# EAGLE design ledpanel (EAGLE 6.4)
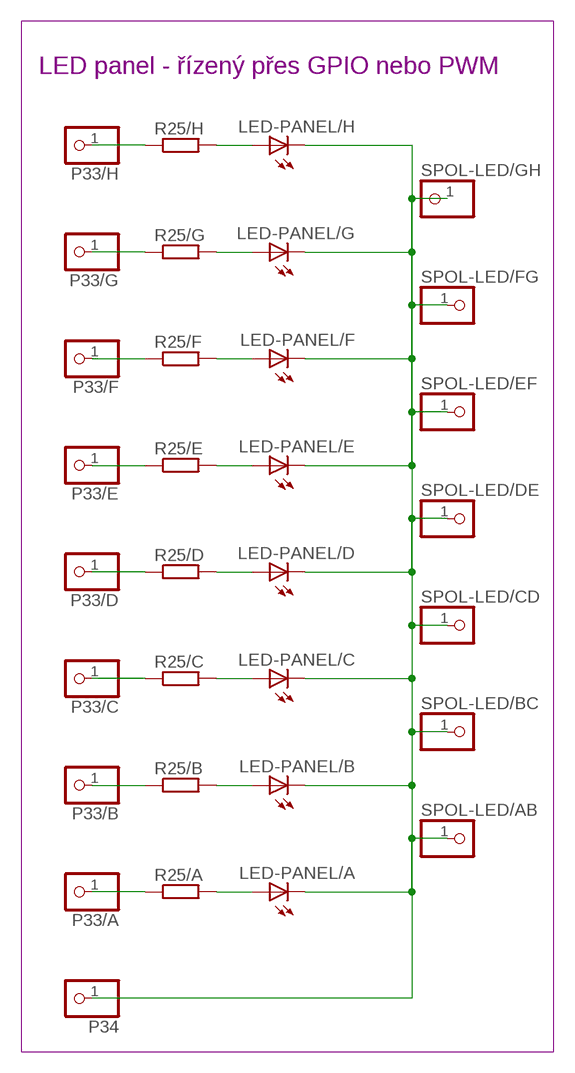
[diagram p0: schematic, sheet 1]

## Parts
LED-PANEL/A  TLLG4400  [LED3MM]
LED-PANEL/B  TLLG4400  [LED3MM]
LED-PANEL/C  TLLG4400  [LED3MM]
LED-PANEL/D  TLLG4400  [LED3MM]
LED-PANEL/E  TLLG4400  [LED3MM]
LED-PANEL/F  TLLG4400  [LED3MM]
LED-PANEL/G  TLLG4400  [LED3MM]
LED-PANEL/H  TLLG4400  [LED3MM]
P33/A  HEADER-1X1  [1X01_OVAL]
P33/B  HEADER-1X1  [1X01_OVAL]
P33/C  HEADER-1X1  [1X01_OVAL]
P33/D  HEADER-1X1  [1X01_OVAL]
P33/E  HEADER-1X1  [1X01_OVAL]
P33/F  HEADER-1X1  [1X01_OVAL]
P33/G  HEADER-1X1  [1X01_OVAL]
P33/H  HEADER-1X1  [1X01_OVAL]
P34  HEADER-1X1  [1X01_OVAL]
R25/A  1k  R-EU_M0805  [M0805]
R25/B  1k  R-EU_M0805  [M0805]
R25/C  1k  R-EU_M0805  [M0805]
R25/D  1k  R-EU_M0805  [M0805]
R25/E  1k  R-EU_M0805  [M0805]
R25/F  1k  R-EU_M0805  [M0805]
R25/G  1k  R-EU_M0805  [M0805]
R25/H  1k  R-EU_M0805  [M0805]
SPOL-LED/AB  PINHD-1X1  [1X01]
SPOL-LED/BC  PINHD-1X1  [1X01]
SPOL-LED/CD  PINHD-1X1  [1X01]
SPOL-LED/DE  PINHD-1X1  [1X01]
SPOL-LED/EF  PINHD-1X1  [1X01]
SPOL-LED/FG  PINHD-1X1  [1X01]
SPOL-LED/GH  PINHD-1X1  [1X01]

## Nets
LED-SPOL: LED-PANEL/A.K(C) LED-PANEL/B.K(C) LED-PANEL/C.K(C) LED-PANEL/D.K(C) LED-PANEL/E.K(C) LED-PANEL/F.K(C) LED-PANEL/G.K(C) LED-PANEL/H.K(C) P34.1 SPOL-LED/AB.1 SPOL-LED/BC.1 SPOL-LED/CD.1 SPOL-LED/DE.1 SPOL-LED/EF.1 SPOL-LED/FG.1 SPOL-LED/GH.1
PRA: P33/A.1 R25/A.1
PRB: P33/B.1 R25/B.1
PRC: P33/C.1 R25/C.1
PRD: P33/D.1 R25/D.1
PRE: P33/E.1 R25/E.1
PRF: P33/F.1 R25/F.1
PRG: P33/G.1 R25/G.1
PRH: P33/H.1 R25/H.1
RLA: LED-PANEL/A.A R25/A.2
RLB: LED-PANEL/B.A R25/B.2
RLC: LED-PANEL/C.A R25/C.2
RLD: LED-PANEL/D.A R25/D.2
RLE: LED-PANEL/E.A R25/E.2
RLF: LED-PANEL/F.A R25/F.2
RLG: LED-PANEL/G.A R25/G.2
RLH: LED-PANEL/H.A R25/H.2

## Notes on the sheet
- LED panel - řízený přes GPIO nebo PWM

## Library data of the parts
LED-PANEL/A LED-PANEL/B LED-PANEL/C LED-PANEL/D LED-PANEL/E LED-PANEL/F LED-PANEL/G LED-PANEL/H = led:TLLG4400: Low Current (2mA) LED 3 mm Tinted Diffused Package color GREEN; MF: VISHAY SEMICONDUCTOR; OC_FARNELL: 1612435
P33/A P33/B P33/C P33/D P33/E P33/F P33/G P33/H P34 = nonolith:HEADER-1X1: PIN HEADER
R25/A R25/B R25/C R25/D R25/E R25/F R25/G R25/H = resistor:R-EU_: RESISTOR, European symbol
SPOL-LED/AB SPOL-LED/BC SPOL-LED/CD SPOL-LED/DE SPOL-LED/EF SPOL-LED/FG SPOL-LED/GH = pinhead:PINHD-1X1: PIN HEADER

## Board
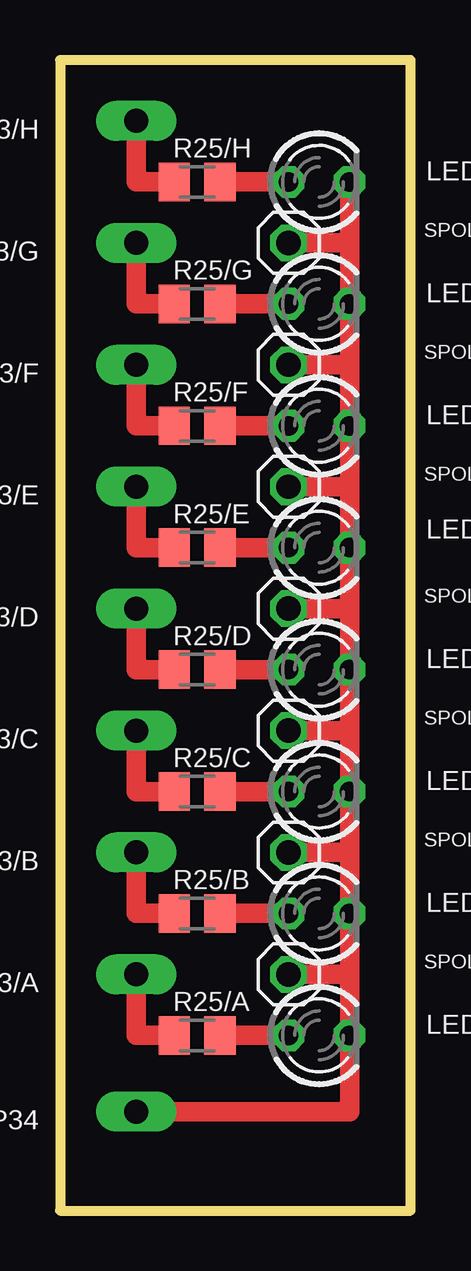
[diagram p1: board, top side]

Size 14.61 x 47.94 mm. Coordinates in mm from the lower left corner, seen from the top.
Outline: 0,0 14.61,0 14.61,47.94 0,47.94 0,0
Copper layers (1*16): Top 0.035mm / dielectric 1.5mm / Bottom 0.035mm
Design rules "default": minimum track width 10mil, minimum drill 24mil, track to track 8mil, track to pad 8mil, pad to pad 8mil, via to via 8mil, smd to smd 8mil, copper to edge 40mil, drill to drill 8mil, minimum pad ring 10mil, minimum via ring 8mil, stop-mask expansion 4mil, vias tented up to drill 0mil, thermal gap 10mil

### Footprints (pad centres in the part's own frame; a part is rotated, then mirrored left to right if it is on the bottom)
LED3MM = drill 0.813 octagon: A -1.27,0; K 1.27,0
1X01_OVAL = drill 1 pad 1.676 long: 1 0,0
M0805 = smd 1.3 x 1.6: 1 -0.95,0; 2 0.95,0
1X01 = drill 1.016 octagon: 1 0,0

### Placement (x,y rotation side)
LED-PANEL/A  10.79,7.3 0 top
LED-PANEL/B  10.79,12.38 0 top
LED-PANEL/C  10.79,17.46 0 top
LED-PANEL/D  10.79,22.54 0 top
LED-PANEL/E  10.79,27.62 0 top
LED-PANEL/F  10.79,32.7 0 top
LED-PANEL/G  10.79,37.78 0 top
LED-PANEL/H  10.79,42.86 0 top
P33/A  3.17,9.84 90 top
P33/B  3.17,14.92 90 top
P33/C  3.17,20 90 top
P33/D  3.17,25.08 90 top
P33/E  3.17,30.16 90 top
P33/F  3.17,35.24 90 top
P33/G  3.17,40.32 270 top
P33/H  3.17,45.4 90 top
P34  3.17,4.13 90 top
R25/A  5.71,7.3 0 top
R25/B  5.71,12.38 0 top
R25/C  5.71,17.46 0 top
R25/D  5.71,22.54 0 top
R25/E  5.71,27.62 0 top
R25/F  5.71,32.7 0 top
R25/G  5.71,37.78 0 top
R25/H  5.71,42.86 0 top
SPOL-LED/AB  9.53,9.84 0 top
SPOL-LED/BC  9.53,14.92 0 top
SPOL-LED/CD  9.53,20 0 top
SPOL-LED/DE  9.53,25.08 0 top
SPOL-LED/EF  9.53,30.16 0 top
SPOL-LED/FG  9.53,35.24 0 top
SPOL-LED/GH  9.53,40.32 0 top

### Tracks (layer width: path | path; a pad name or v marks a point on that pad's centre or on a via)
LED-SPOL
  Top 0.813: LED-PANEL/H.K 12.07,40.32 | 12.07,40.32 LED-PANEL/G.K 12.07,35.24 | 12.07,35.24 LED-PANEL/F.K 12.07,30.16 | 12.07,30.16 LED-PANEL/E.K 12.07,25.08 | 12.07,25.08 LED-PANEL/D.K 12.07,20 | 12.07,20 LED-PANEL/C.K 12.07,14.92 | 12.07,14.92 LED-PANEL/B.K 12.07,9.84 | 12.07,9.84 LED-PANEL/A.K 12.07,4.13 P34.1 | SPOL-LED/AB.1 12.07,9.84 | SPOL-LED/BC.1 12.07,14.92 | SPOL-LED/CD.1 12.07,20 | SPOL-LED/DE.1 12.07,25.08 | SPOL-LED/EF.1 12.07,30.16 | SPOL-LED/FG.1 12.07,35.24 | SPOL-LED/GH.1 12.07,40.32
PRA
  Top 0.813: R25/A.1 3.17,7.3 P33/A.1
PRB
  Top 0.813: R25/B.1 3.17,12.38 P33/B.1
PRC
  Top 0.813: R25/C.1 3.17,17.46 P33/C.1
PRD
  Top 0.813: R25/D.1 3.17,22.54 P33/D.1
PRE
  Top 0.813: R25/E.1 3.17,27.62 P33/E.1
PRF
  Top 0.813: R25/F.1 3.17,32.7 P33/F.1
PRG
  Top 0.813: R25/G.1 3.17,37.78 P33/G.1
PRH
  Top 0.813: R25/H.1 3.17,42.86 P33/H.1
RLA
  Top 0.813: LED-PANEL/A.A R25/A.2
RLB
  Top 0.813: LED-PANEL/B.A R25/B.2
RLC
  Top 0.813: LED-PANEL/C.A R25/C.2
RLD
  Top 0.813: LED-PANEL/D.A R25/D.2
RLE
  Top 0.813: LED-PANEL/E.A R25/E.2
RLF
  Top 0.813: LED-PANEL/F.A R25/F.2
RLG
  Top 0.813: LED-PANEL/G.A R25/G.2
RLH
  Top 0.813: LED-PANEL/H.A R25/H.2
